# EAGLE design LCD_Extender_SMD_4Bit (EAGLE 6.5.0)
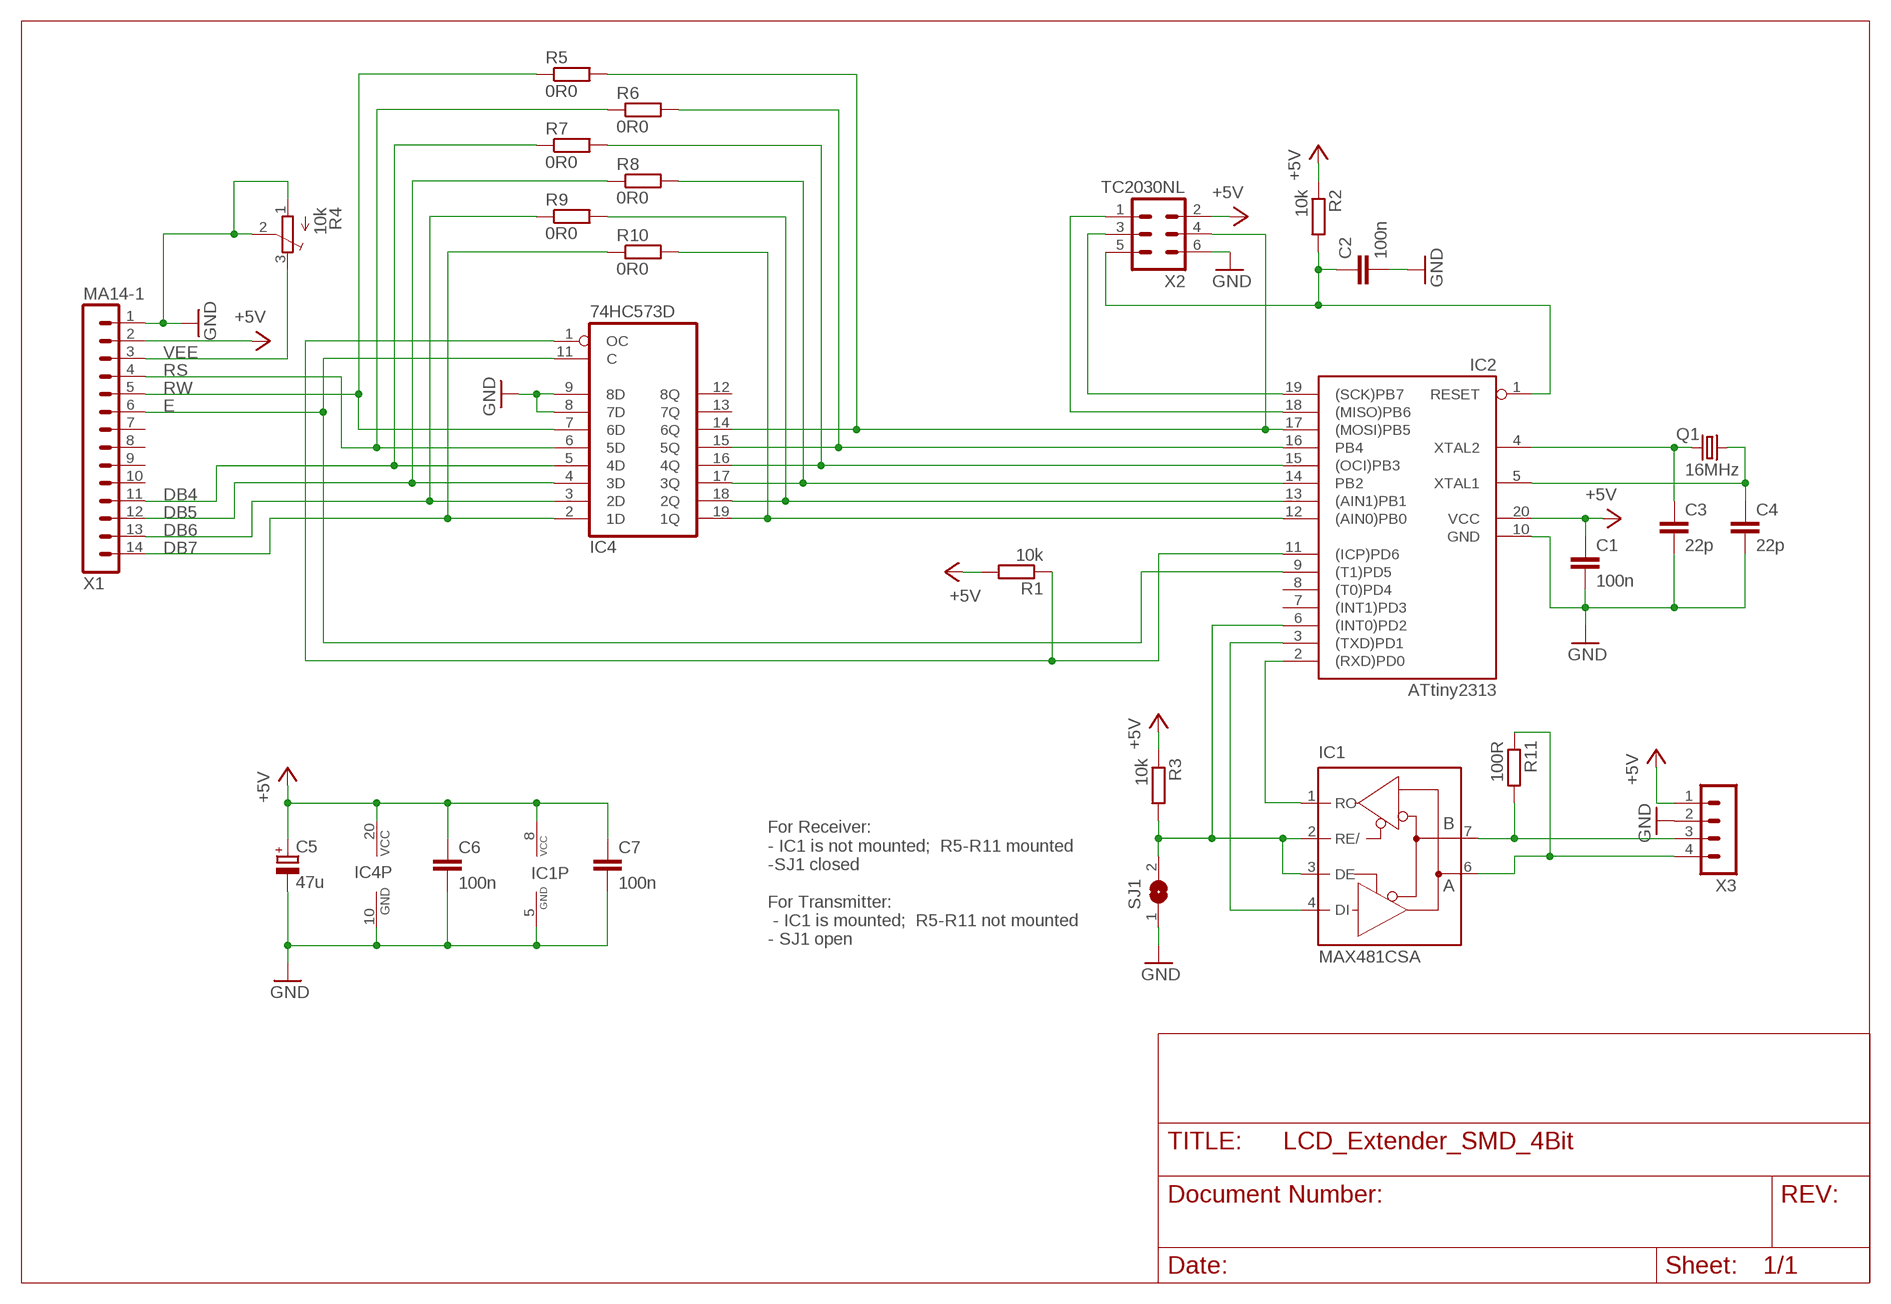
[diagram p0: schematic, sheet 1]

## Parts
C1  100n  C-EUC1206  [C1206]
C2  100n  C-EUC1206  [C1206]
C3  22p  C-EUC1206  [C1206]
C4  22p  C-EUC1206  [C1206]
C5  47u  CPOL-EUCT3528  [CT3528]
C6  100n  C-EUC1206  [C1206]
C7  100n  C-EUC1206  [C1206]
IC1  MAX481CSA  [SO08]
IC2  ATtiny2313  AT90S2313S  [SO20L]
IC4  74HC573D  [SO20W]
Q1  16MHz  CRYSTALHC49UP  [HC49UP]
R1  10k  R-EU_R1206  [R1206]
R2  10k  R-EU_R1206  [R1206]
R3  10k  R-EU_R1206  [R1206]
R4  10k  TRIM_EU-3223G  [3223G]
R5  0R0  R-EU_R0603  [R0603]
R6  0R0  R-EU_R0603  [R0603]
R7  0R0  R-EU_R0603  [R0603]
R8  0R0  R-EU_R0603  [R0603]
R9  0R0  R-EU_R0603  [R0603]
R10  0R0  R-EU_R0603  [R0603]
R11  100R  R-EU_R1206  [R1206]
SJ1  SJ  [SJ]
X1  MA14-1  [MA14-1]
X2  TC2030NL  [TC2030-IDC-NL]
X3  MA04-1  [MA04-1]

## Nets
+5V: C1.1 C5.+ C6.1 C7.1 IC1.8(VCC) IC2.20(VCC) IC4.20(VCC) R1.2 R2.1 R3.1 X1.2 X2.2 X3.1
DB4: IC4.5(4D) R7.1 X1.11
DB5: IC4.4(3D) R8.1 X1.12
DB6: IC4.3(2D) R9.1 X1.13
DB7: IC4.2(1D) R10.1 X1.14
E: IC2.9((T1)PD5) IC4.11(C) X1.6
GND: C1.2 C2.2 C3.2 C4.2 C5.- C6.2 C7.2 IC1.5(GND) IC2.10(GND) IC4.8(7D) IC4.9(8D) IC4.10(GND) R4.1(A) R4.2(S) SJ1.1 X1.1 X2.6 X3.2
N$1: IC2.17((MOSI)PB5) IC4.14(6Q) R5.2 X2.4
N$2: C3.1 IC2.4(XTAL2) Q1.1
N$3: IC2.15((OCI)PB3) IC4.16(4Q) R7.2
N$4: IC2.16(PB4) IC4.15(5Q) R6.2
N$5: IC2.18((MISO)PB6) X2.1
N$7: IC1.4(DI) IC2.3((TXD)PD1)
N$9: C4.1 IC2.5(XTAL1) Q1.2
N$10: IC1.7(B) R11.2 X3.3
N$11: IC1.6(A) R11.1 X3.4
N$14: C2.1 IC2.1(RESET) R2.2 X2.5
N$15: IC2.11((ICP)PD6) IC4.1(OC) R1.1
N$23: IC2.19((SCK)PB7) X2.3
N$25: IC2.12((AIN0)PB0) IC4.19(1Q) R10.2
N$26: IC2.13((AIN1)PB1) IC4.18(2Q) R9.2
N$27: IC2.14(PB2) IC4.17(3Q) R8.2
N$29: IC1.1(RO) IC2.2((RXD)PD0)
N$30: IC1.2(RE/) IC1.3(DE) IC2.6((INT0)PD2) R3.2 SJ1.2
RS: IC4.6(5D) R6.1 X1.4
RW: IC4.7(6D) R5.1 X1.5
VEE: R4.3(E) X1.3
Unconnected: IC2.7((INT1)PD3) IC2.8((T0)PD4) IC4.12(8Q) IC4.13(7Q) X1.7 X1.8 X1.9 X1.10

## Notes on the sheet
- For Receiver:
  - IC1 is not mounted;  R5-R11 mounted
  -SJ1 closed
  
  For Transmitter:
   - IC1 is mounted;  R5-R11 not mounted
  - SJ1 open

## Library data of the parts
C1-C4 C6 C7 = rcl:C-EU: CAPACITOR, European symbol
C5 = rcl:CPOL-EU: POLARIZED CAPACITOR, European symbol
IC1 = maxim:MAX481CSA: RS485 TRANSEIVER; MF: MAXIM; MPN: MAX481CSA; OC_FARNELL: unknown; OC_NEWARK: 90C3817
IC2 = atmel:AT90S2313: MICROCONTROLLER 2 Kbytes FLASH 128 bytes SRAM 128 bytes EEPROM UART; OC_FARNELL: unknown; OC_NEWARK: unknown
IC4 = 74xx-eu:74*573: 8-bit D latch BUS DRIVER
Q1 = crystal:CRYSTAL: CRYSTAL; OC_FARNELL: unknown; OC_NEWARK: unknown
R1-R3 R5-R11 = rcl:R-EU_: RESISTOR, European symbol
R4 = pot:TRIM_EU-: POTENTIOMETER
SJ1 = jumper:SJ: SMD solder JUMPER
X1 = Brunner:MA14-1
X2 = Brunner:TC2030
X3 = con-lstb:MA04-1: PIN HEADER; OC_FARNELL: unknown; OC_NEWARK: unknown

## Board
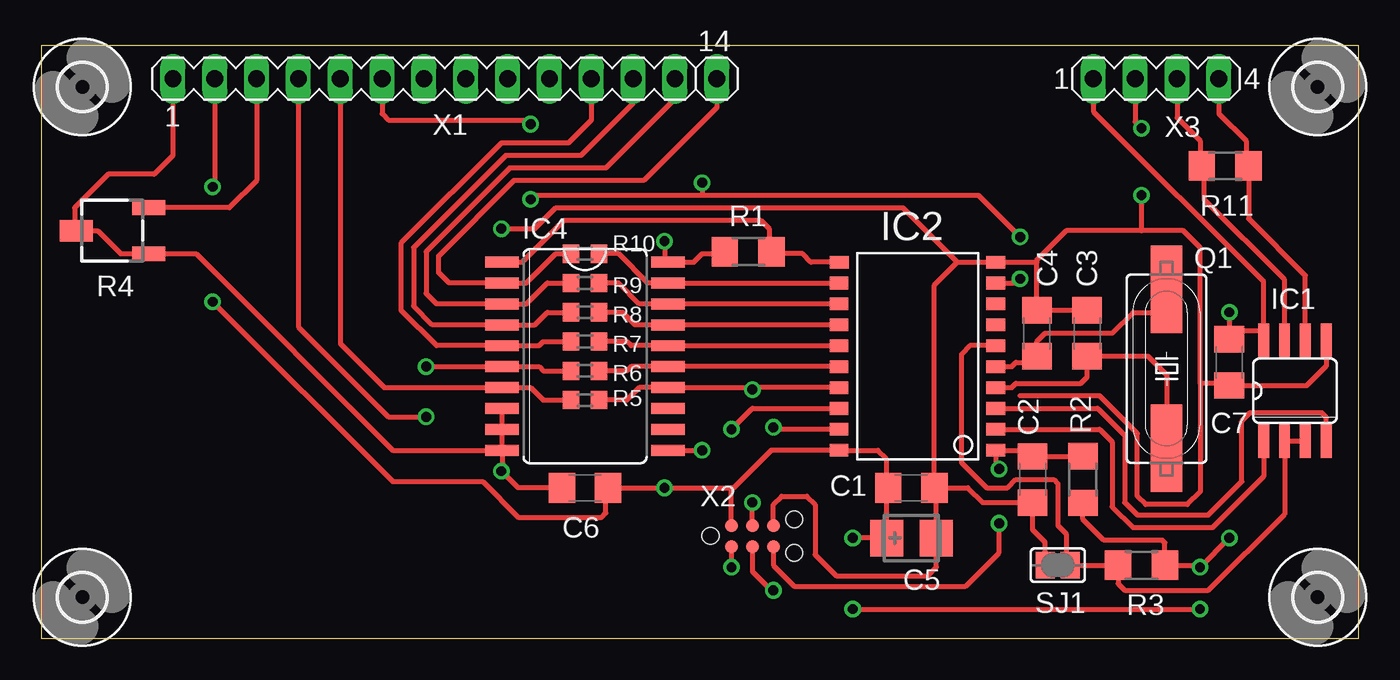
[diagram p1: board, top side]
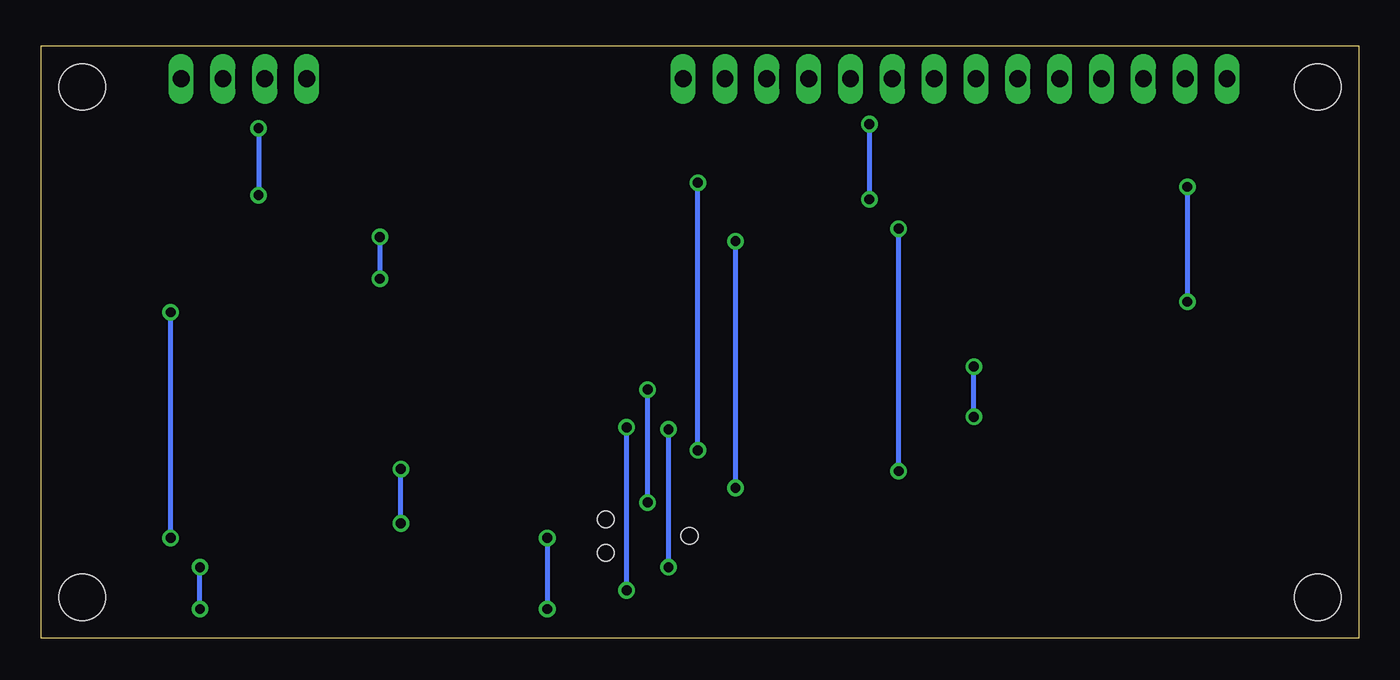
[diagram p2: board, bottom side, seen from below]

Size 80 x 36 mm. Coordinates in mm from the lower left corner, seen from the top.
Outline: 0,36 0,0 80,0 80,36 0,36
Copper layers (1*16): Top 0.035mm / dielectric 1.5mm / Bottom 0.035mm
Design rules "default *": minimum track width 10mil, minimum drill 0.6mm, track to track 0.3mm, track to pad 0.3mm, pad to pad 0.3mm, via to via 0.3mm, smd to smd 8mil, copper to edge 0.4mm, drill to drill 8mil, minimum pad ring 10mil, minimum via ring 8mil, stop-mask expansion 4mil, vias tented up to drill 0mil, thermal gap 10mil

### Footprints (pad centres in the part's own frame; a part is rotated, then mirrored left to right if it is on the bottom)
C1206 = smd 1.6 x 1.8: 1 -1.4,0; 2 1.4,0
CT3528 = smd 2 x 2.2: + -1.5,0; - 1.5,0
SO08 = smd 0.66 x 2.032: 1 -1.905,-3.073; 2 -0.635,-3.073; 3 0.635,-3.073; 4 1.905,-3.073; 5 1.905,3.073; 6 0.635,3.073; 7 -0.635,3.073; 8 -1.905,3.073
SO20L = smd 0.762 x 1.143: 1 -5.08,-5.131; 2 -3.81,-5.131; 3 -2.54,-5.131; 4 -1.27,-5.131; 5 0,-5.131; 6 1.27,-5.131; 7 2.54,-5.131; 8 3.81,-5.131; 9 5.08,-5.131; 10 6.35,-5.131; 11 6.35,4.369; 12 5.08,4.394; 13 3.81,4.394; 14 2.54,4.394; 15 1.27,4.394; 16 0,4.394; 17 -1.27,4.394; 18 -2.54,4.394; 19 -3.81,4.394; 20 -5.08,4.394
SO20W = smd 0.66 x 2.032: 1 -5.715,-5.029; 2 -4.445,-5.029; 3 -3.175,-5.029; 4 -1.905,-5.029; 5 -0.635,-5.029; 6 0.635,-5.029; 7 1.905,-5.029; 8 3.175,-5.029; 9 4.445,-5.029; 10 5.715,-5.029; 11 5.715,5.029; 12 4.445,5.029; 13 3.175,5.029; 14 1.905,5.029; 15 0.635,5.029; 16 -0.635,5.029; 17 -1.905,5.029; 18 -3.175,5.029; 19 -4.445,5.029; 20 -5.715,5.029
HC49UP = smd 5.334 x 1.93: 1 -4.826,0; 2 4.826,0
R1206 = smd 1.6 x 1.803: 1 -1.422,0; 2 1.422,0
3223G = smd 2 x 0.9: 1 -2.2,1.4; 3 -2.2,-1.4 | smd 2 x 1.3: 2 2.2,0
R0603 = smd 1 x 1.1: 1 -0.85,0; 2 0.85,0
SJ = smd 1.168 x 1.6: 1 -0.762,0; 2 0.762,0
2,8 = hole 2.8: 0,0
MA14-1 = drill 1.016 long: 1 -16.51,0; 2 -13.97,0; 3 -11.43,0; 4 -8.89,0; 5 -6.35,0; 6 -3.81,0; 7 -1.27,0; 8 1.27,0; 9 3.81,0; 10 6.35,0; 11 8.89,0; 12 11.43,0; 13 13.97,0; 14 16.51,0
TC2030-IDC-NL = smd 0.78 x 0.78: 1 -1.27,-0.635; 2 -1.27,0.635; 3 0,-0.635; 4 0,0.635; 5 1.27,-0.635; 6 1.27,0.635 | hole 1: -2.54,0; 2.54,1.016; 2.54,-1.016
MA04-1 = drill 1.016 long: 1 -3.81,0; 2 -1.27,0; 3 1.27,0; 4 3.81,0

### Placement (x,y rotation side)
C1  52.83,9.14 0 top
C2  60.2,9.65 270 top
C3  63.5,18.54 90 top
C4  60.45,18.54 90 top
C5  52.83,6.1 0 top
C6  33.02,9.14 180 top
C7  72.14,16.76 270 top
IC1  76.12,15.04 0 top
IC2  52.83,16.51 90 top
IC4  33.02,17.14 270 top
Q1  68.33,16.38 90 top
R1  42.93,23.5 180 top
R2  63.25,9.65 90 top
R3  66.8,4.45 180 top
R4  4.32,24.77 180 top
R5  33.02,14.48 0 top
R6  33.02,16.26 0 top
R7  33.02,18.03 0 top
R8  33.02,19.81 0 top
R9  33.02,21.59 0 top
R10  33.02,23.37 0 top
R11  71.88,28.7 180 top
SJ1  61.72,4.45 0 top
U$1  [2,8]  2.5,33.5 0 top
U$2  [2,8]  2.5,2.5 0 top
U$3  [2,8]  77.5,2.5 0 top
U$4  [2,8]  77.5,33.5 0 top
X1  24.51,34 0 top
X2  43.18,6.22 0 top
X3  67.69,34 0 top

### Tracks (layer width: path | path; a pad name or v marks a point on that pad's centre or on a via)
+5V  (via drill 0.6)
  Top 0.305: 34.29,9.27 C6.1 | C6.1 v37.85,9.14 41.91,9.14 | 41.91,9.14 42.04,9.14 44.32,11.43 IC2.20 50.8,11.43 51.31,10.92 51.31,9.27 C1.1 51.33,9.04 C5.+ v49.28,6.1 | 63.25,8.48 R2.1 63.25,7.24 64.52,5.97 68.07,5.97 68.22,5.82 R3.1 70.23,4.45 v70.36,4.32 v72.14,6.1 | v72.14,19.81 C7.1 72.64,18.67 74.17,18.67 74.22,18.62 IC1.8 74.22,21.67 63.88,32 X3.1 | v10.41,20.45 21.34,9.53 26.8,9.53 28.96,7.37 34.04,7.37 34.29,7.62 34.29,9.01 C6.1 | X2.2 41.91,9.14 | R1.2 41.38,23.37 40.13,23.37 39.62,22.86 IC4.20 37.85,23.06 v37.85,24.13 | X1.2 10.54,27.56 v10.41,27.43 | v49.28,1.78 v70.36,1.78
  Bottom 0.305: v37.85,24.13 v37.85,9.14 | v10.41,27.43 v10.41,20.45 | v49.28,6.1 v49.28,1.78 | v70.36,1.78 v70.36,4.32 | v72.14,6.1 v72.14,19.81
DB4
  Top 0.305: X1.11 33.4,31.5 32,30.1 27.94,30.1 21.84,24 21.84,19.94 24,17.78 IC4.5 30.23,17.78 30.48,18.03 R7.1
DB5
  Top 0.305: X1.12 35.94,32.51 32.77,29.34 28.19,29.34 22.61,23.75 22.61,20.19 23.75,19.05 IC4.4 29.97,19.05 30.73,19.81 R8.1
DB6
  Top 0.305: X1.13 38.48,32.77 34.29,28.57 28.45,28.57 23.37,23.5 23.37,20.95 24,20.32 IC4.3 29.46,20.32 30.73,21.59 R9.1
DB7
  Top 0.305: X1.14 41.02,32.26 36.58,27.81 28.7,27.81 24.13,23.24 24.13,22.23 24.77,21.59 IC4.2 29.46,21.59 31.24,23.37 R10.1
E  (via drill 0.6)
  Top 0.305: X1.6 20.7,31.88 21.08,31.5 29.46,31.5 v29.72,31.24 | v29.72,26.67 29.97,26.92 40.13,26.92 | 40.13,26.92 56.9,26.92 v59.44,24.38 | IC2.9 59.18,21.59 v59.44,21.84 | IC4.11 v40.13,11.43 | v40.13,27.69 40.13,26.92
  Bottom 0.305: v29.72,31.24 v29.72,26.67 | v59.44,24.38 v59.44,21.84 | v40.13,11.43 v40.13,27.69
GND  (via drill 0.6)
  Top 0.305: C1.2 54.23,21.47 55.63,22.86 | 55.63,22.86 IC2.10 60.45,22.86 | C3.2 C4.2 60.45,22.86 | C1.2 56.26,9.14 57.15,8.25 C2.2 60.2,6.6 60.96,5.84 SJ1.1 | 55.63,22.86 52.32,26.16 31.24,26.16 29.97,24.89 v27.94,24.89 | 66.8,24.77 69.34,24.77 70.36,23.75 70.36,15.49 | 66.8,24.77 62.23,24.77 60.45,22.99 60.45,22.86 | X1.1 8,29.34 6.86,28.19 4.06,28.19 2.03,26.16 2.03,24.85 R4.2 3.43,24.77 4.83,23.37 R4.1 9.4,23.36 21.34,11.43 IC4.10 | 59.44,14.73 64.26,14.73 66.55,12.45 66.55,8.64 67.06,8.13 69.6,8.13 70.36,8.89 70.36,15.49 | IC1.5 78.03,16.56 76.83,15.36 C7.2 72.01,15.49 70.36,15.49 | IC4.10 27.99,10.21 v27.94,10.16 28.96,9.14 C6.2 | X3.2 66.42,31.37 v66.8,30.99 | v66.8,26.92 66.8,24.77 | IC4.10 IC4.9 IC4.8 | X2.6 44.45,8.13 44.96,8.64 46.48,8.64 46.99,8.13 46.99,5.08 48.26,3.81 53.85,3.81 54.36,4.32 54.36,6.07 C5.- 54.33,9.04 C1.2
  Bottom 0.305: v27.94,10.16 v27.94,24.89 | v66.8,30.99 v66.8,26.92
N$1  (via drill 0.6)
  Top 0.305: X2.4 v43.18,8.26 | IC2.17 43.31,15.24 v43.18,15.11 43.05,15.24 IC4.14 36.32,15.24 35.56,14.48 R5.2
  Bottom 0.305: v43.18,8.26 v43.18,15.11
N$2
  Top 0.305: IC2.4 58.93,15.24 59.18,15.49 63.12,15.49 63.5,15.88 C3.1 67.19,17.14 68.33,16 Q1.1
N$3
  Top 0.305: IC2.15 IC4.16 35.81,17.78 35.56,18.03 R7.2
N$4
  Top 0.305: IC2.16 IC4.15 35.81,16.51 35.56,16.26 R6.2
N$5  (via drill 0.6)
  Top 0.305: X2.1 v41.91,4.32 | v41.91,12.7 43.18,13.97 IC2.18
  Bottom 0.305: v41.91,4.32 v41.91,12.7
N$7
  Top 0.305: IC2.3 64.14,13.97 65.79,12.32 65.79,8.26 66.55,7.49 70.87,7.49 72.9,9.53 72.9,13.21 73.41,13.72 77.72,13.72 78.03,13.41 IC1.4
N$9
  Top 0.305: Q1.2 68.33,20.32 67.82,19.81 66.29,19.81 65.02,18.54 60.96,18.54 60.45,18.03 C4.1 60.07,16.76 59.18,16.76 58.93,16.51 IC2.5
N$10
  Top 0.305: IC1.7 75.49,21.79 70.61,26.67 70.61,28.55 R11.2 70.36,28.8 70.36,30.23 68.96,31.62 X3.3
N$11
  Top 0.305: X3.4 71.5,31.88 73.15,30.23 73.15,28.85 R11.1 73.3,25.5 76.76,22.05 IC1.6
N$14  (via drill 0.6)
  Top 0.305: X2.5 44.45,4.45 45.72,3.17 56.13,3.17 58.17,5.21 v58.17,6.99 | v58.17,10.29 57.96,10.49 IC2.1 59.82,11.43 C2.1 63.22,11.05 R2.2
  Bottom 0.305: v58.17,6.99 v58.17,10.29
N$15
  Top 0.305: IC4.1 29.21,22.86 31.75,25.4 43.69,25.4 44.2,24.89 44.2,23.65 R1.1 44.48,23.37 46.23,23.37 46.74,22.86 IC2.11
N$23  (via drill 0.6)
  Top 0.305: X2.3 43.18,4.06 44.32,2.92 v44.45,2.92 | IC2.19 44.58,12.7 v44.45,12.83 44.32,12.7
  Bottom 0.305: v44.45,2.92 v44.45,12.83
N$25
  Top 0.305: IC2.12 IC4.19 36.83,21.59 35.05,23.37 R10.2
N$26
  Top 0.305: IC2.13 IC4.18 36.32,20.32 35.05,21.59 R9.2
N$27
  Top 0.305: IC2.14 IC4.17 36.07,19.05 35.31,19.81 R8.2
N$29
  Top 0.305: IC1.1 74.22,9.83 71.12,6.73 66.29,6.73 65.02,8 65.02,11.94 64.26,12.7 IC2.2
N$30
  Top 0.305: IC1.3 IC1.2 75.49,7.54 70.87,2.92 65.79,2.92 65.38,3.33 R3.2 SJ1.2 62.23,4.7 62.23,6.35 61.72,6.86 61.72,9.4 61.47,9.65 59.18,9.65 58.67,9.14 57.4,9.14 55.88,10.67 55.88,17.27 56.39,17.78 IC2.6
RS  (via drill 0.6)
  Top 0.305: R6.1 30.48,16.26 30.23,16.51 IC4.6 v23.37,16.51 | X1.4 15.62,18.92 21.08,13.46 v23.37,13.46
  Bottom 0.305: v23.37,13.46 v23.37,16.51
RW
  Top 0.305: X1.5 18.16,17.91 20.83,15.24 IC4.7 29.72,15.24 30.48,14.48 R5.1
VEE
  Top 0.305: X1.3 13.08,27.81 11.43,26.16 R4.3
